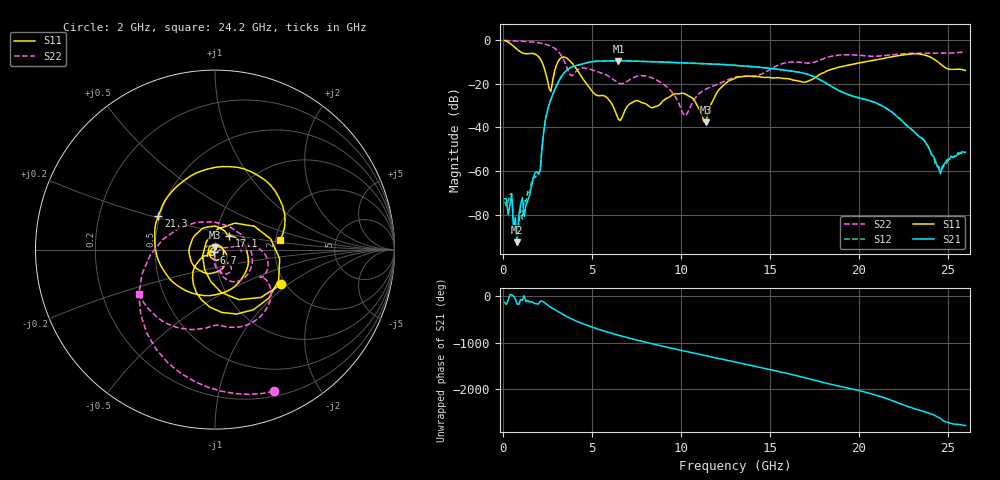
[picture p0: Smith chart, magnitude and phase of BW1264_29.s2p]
!Keysight Technologies,N5245B,MY57181159,A.13.60.06
!Date: Friday, December 18, 2020 23:53:28
!Correction: S11(Full 2 Port(1,2))
!S21(Full 2 Port(1,2))
!S12(Full 2 Port(1,2))
!S22(Full 2 Port(1,2))
!S2P File: Measurements: S11, S21, S12, S22:
# Hz S  dB  R 50
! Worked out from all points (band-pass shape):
!   260 points, 100 MHz to 26 GHz, reference 50 ohm
!   highest |S21| = -9.61 dB at 6.5 GHz (marker M1); lowest = -92.5 dB at 800 MHz (marker M2)
!   |S21| within 3 dB of the highest: 3.829 GHz to 14.52 GHz (10.69 GHz wide, 117 % of centre)
!   lowest |S11| = -37.7 dB at 11.4 GHz (marker M3), VSWR 1.03, Z = 50 + j1.31 ohm
!   |S11| at or under -10 dB: 2.188 GHz to 3.1 GHz (912.7 MHz wide, 34.5 % of centre); 3.816 GHz to 20.4 GHz (16.58 GHz wide, 137 % of centre); 24.44 GHz to end of sweep
!   |S22| runs from -34.6 to -0.3 dB; largest |S21 - S12| = 0.00063
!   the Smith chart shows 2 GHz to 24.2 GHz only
!   S11 on the Smith chart (normalised r, x): 2 GHz: 1.90, -0.89; 6.7 GHz: 0.99, -0.03; 17.1 GHz: 1.16, +0.18; 21.3 GHz: 0.49, +0.21; 24.2 GHz: 2.12, +0.27
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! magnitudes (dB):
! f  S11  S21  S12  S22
! 100 MHz  -0.4  -72.6  -73.9  -0.3
! 300 MHz  -1.1  -79.8  -73.8  -0.4
! 500 MHz  -2.2  -70.7  -70.1  -0.5
! 800 MHz  -4.3  -92.5  -94.2  -0.6
! 2 GHz  -7.6  -61.4  -61.2  -1.4
! 2.4 GHz  -15.0  -36.3  -36.4  -2.0
! 2.8 GHz  -18.8  -25.1  -25.1  -3.3
! 3.4 GHz  -7.9  -15.6  -15.6  -8.8
! 4.5 GHz  -17.8  -11.0  -11.0  -12.8
! 6.5 GHz  -36.3  -9.6  -9.6  -19.8
! 6.7 GHz  -35.4  -9.6  -9.6  -20.1
! 8.8 GHz  -29.7  -10.1  -10.1  -19.1
! 10.2 GHz  -24.5  -10.5  -10.5  -34.6
! 11.4 GHz  -37.7  -10.9  -10.9  -22.6
! 13.1 GHz  -17.4  -11.7  -11.7  -17.1
! 17.1 GHz  -19.1  -15.7  -15.7  -10.6
! 17.4 GHz  -18.0  -16.5  -16.5  -10.4
! 21.3 GHz  -8.7  -30.1  -30.1  -7.3
! 21.7 GHz  -8.0  -32.1  -32.1  -7.0
! 24.2 GHz  -8.7  -53.2  -53.1  -6.1
! 24.6 GHz  -11.1  -61.2  -59.8  -6.1
! 26 GHz  -14.0  -51.3  -51.6  -5.5
